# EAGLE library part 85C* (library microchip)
Serial EEPROM 1 K/2 K/4 K, 5.0 V, CMOS 85C72/82/92
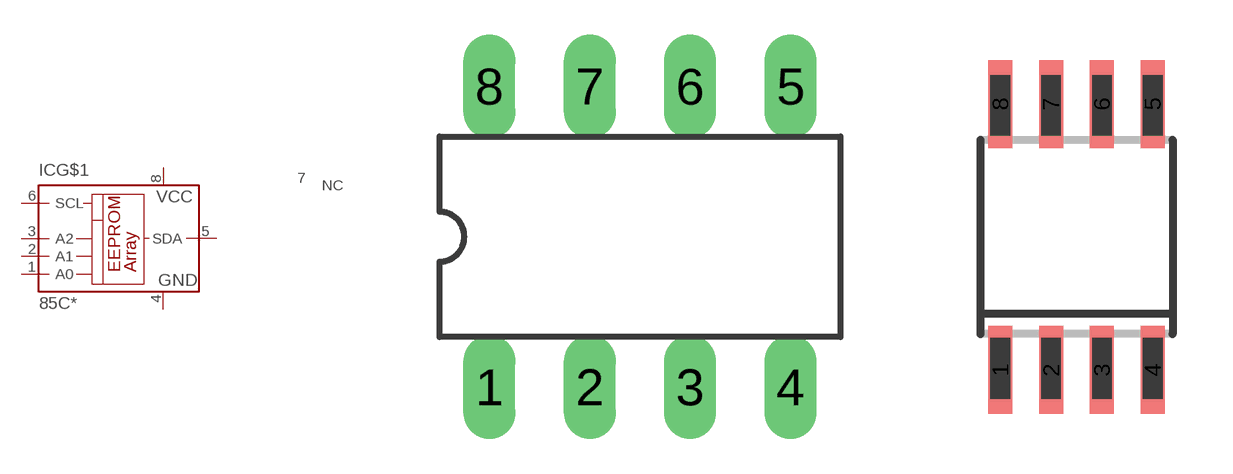
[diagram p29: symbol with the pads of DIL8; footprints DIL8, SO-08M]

Designator prefix IC; gates G$1=85C72 7=NC

## 85C72P (OC_FARNELL: unknown; OC_NEWARK: unknown), 85C82P (OC_FARNELL: unknown; OC_NEWARK: unknown), 85C92P (OC_FARNELL: unknown; OC_NEWARK: unknown)  [DIL8]
1  G$1:A0  in
2  G$1:A1  in
3  G$1:A2  in
4  G$1:GND  pwr
5  G$1:SDA  hiz
6  G$1:SCL  in
7  7:NC  nc
8  G$1:VCC  pwr

## 85CSM (OC_FARNELL: unknown; OC_NEWARK: unknown), 85C72SM (OC_FARNELL: unknown; OC_NEWARK: unknown), 85C82SM (OC_FARNELL: unknown; OC_NEWARK: unknown), 85C92SM (OC_FARNELL: unknown; OC_NEWARK: unknown)  [SO-08M]
Pads as for DIL8

## Footprint DIL8 (pad centres in mm)
Dual In Line package type P
drill 0.813 long: 1 -3.81,-3.81; 2 -1.27,-3.81; 3 1.27,-3.81; 4 3.81,-3.81; 5 3.81,3.81; 6 1.27,3.81; 7 -1.27,3.81; 8 -3.81,3.81

## Footprint SO-08M (pad centres in mm)
Small Outline Medium Plastic Gull Wing 207-mil body, package type SM
smd 0.6 x 2.2: 1 -1.905,-3.33; 2 -0.635,-3.33; 3 0.635,-3.33; 4 1.905,-3.33; 5 1.905,3.33; 6 0.635,3.33; 7 -0.635,3.33; 8 -1.905,3.33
